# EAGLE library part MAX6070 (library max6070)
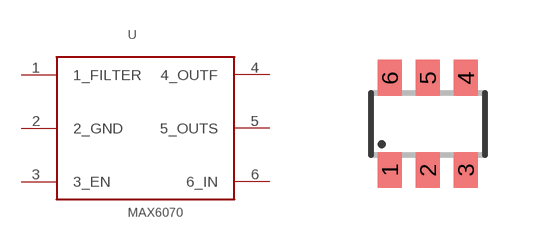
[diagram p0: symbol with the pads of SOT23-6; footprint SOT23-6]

Designator prefix -

## MAX6070  [SOT23-6]
1  1_FILTER  in
2  2_GND  pwr
3  3_EN  in
4  4_OUTF  out
5  5_OUTS  out
6  6_IN  in

## Footprint SOT23-6 (pad centres in mm)
Small Outline Transistor 6 lead
smd 0.6 x 0.9: 1 -0.95,-1.15; 2 0,-1.15; 3 0.95,-1.15; 4 0.95,1.15; 5 0,1.15; 6 -0.95,1.15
